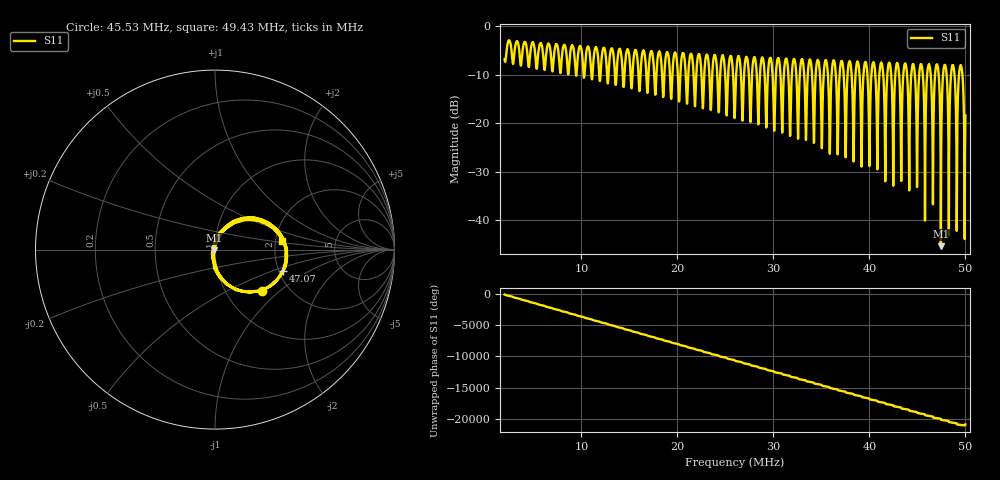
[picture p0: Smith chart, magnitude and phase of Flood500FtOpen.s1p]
! ListType=Lin
!!500FtFloodedOpen
# MHz S RI R 50
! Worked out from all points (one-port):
!   4096 points, 2 MHz to 50 MHz, reference 50 ohm
!   lowest |S11| = -45.3 dB at 47.44 MHz (marker M1), VSWR 1.01, Z = 49.6 - j0.323 ohm
!   |S11| at or under -10 dB: 45.57 MHz to 46.02 MHz (450.4 kHz wide, 0.984 % of centre); 47.22 MHz to 47.67 MHz (454.5 kHz wide, 0.958 % of centre); 48.87 MHz to 49.33 MHz (466.3 kHz wide, 0.95 % of centre)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
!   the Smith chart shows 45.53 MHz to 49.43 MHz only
!   S11 on the Smith chart (normalised r, x): 45.53 MHz: 1.47, -0.76; 47.07 MHz: 2.12, -0.59; 49.43 MHz: 2.17, +0.25
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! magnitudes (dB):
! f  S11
! 2 MHz  -6.8
! 8.001 MHz  -5.5
! 14 MHz  -4.7
! 20 MHz  -8.6
! 26.01 MHz  -16.4
! 32.01 MHz  -7.8
! 36.3 MHz  -7.1
! 36.7 MHz  -26.4
! 37.12 MHz  -7.2
! 37.53 MHz  -27.0
! 38.01 MHz  -7.5
! 40.83 MHz  -29.5
! 41.26 MHz  -7.5
! 41.65 MHz  -32.0
! 42.08 MHz  -7.5
! 42.49 MHz  -32.9
! 42.91 MHz  -7.6
! 43.32 MHz  -31.9
! 43.73 MHz  -7.7
! 44.01 MHz  -13.4
! 45.53 MHz  -9.2
! 46.64 MHz  -30.4
! 47.07 MHz  -8.0
! 47.44 MHz  -45.3
! 47.84 MHz  -8.0
! 48.27 MHz  -35.0
! 49.43 MHz  -8.5
! 50 MHz  -18.4
